(* Logix 5000 AddOnInstructionDefinition export Bronkhorst_FF_Basic_INT_Input; software revision 37.00 *)

ADD_ON_INSTRUCTION Bronkhorst_FF_Basic_INT_Input   (* revision 1.0, vendor Bronkhorst High-Tech B.V. *)
// Extract data from the FLEXI-FLOW Basic INT input connection (in to controller from device)
VAR_IN_OUT
   DataIn : SINT[7]; {required}
END_VAR
VAR_OUTPUT
   Status : USINT; {visible}
   Measure : INT; {visible}
   Pressure_Inlet : INT; {visible}
   Pressure_Outlet : INT; {visible}
END_VAR

ROUTINE Logic   (* structured text *)
   Status := DataIn[0];
   COP(DataIn[1], Measure, 1);
   COP(DataIn[3], Pressure_Inlet, 1);
   COP(DataIn[5], Pressure_Outlet, 1);
END_ROUTINE
END_ADD_ON_INSTRUCTION

ADD_ON_INSTRUCTION Bronkhorst_FF_Basic_INT_Output   (* revision 1.0, vendor Bronkhorst High-Tech B.V. *)
// Fill data for the FLEXI-FLOW Basic INT output connection (out from controller to device)
VAR_IN_OUT
   DataOut : SINT[6]; {required}
END_VAR
VAR_INPUT
   Setpoint : INT; {visible}
   Pressure_Inlet_Setpoint : INT; {visible}
   Pressure_Outlet_Setpoint : INT; {visible}
END_VAR

ROUTINE Logic   (* structured text *)
   COP(Setpoint, DataOut[0], 2);
   COP(Pressure_Inlet_Setpoint, DataOut[2], 2);
   COP(Pressure_Outlet_Setpoint, DataOut[4], 2);
END_ROUTINE
END_ADD_ON_INSTRUCTION
